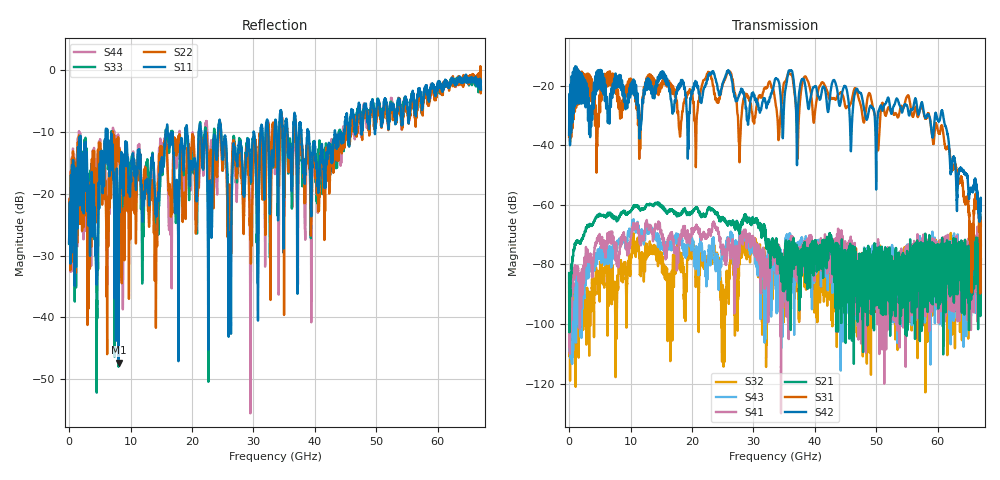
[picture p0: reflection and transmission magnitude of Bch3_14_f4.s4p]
!Agilent Technologies,N5247A,US51170199,A.09.90.13
!Agilent N5247A: A.09.90.13
!Date: Thursday, October 18, 2018 11:10:10
!Correction: S11(Full 4 Port(1,2,3,4))
!S12(Full 4 Port(1,2,3,4))
!S13(Full 4 Port(1,2,3,4))
!S14(Full 4 Port(1,2,3,4))
!S21(Full 4 Port(1,2,3,4))
!S22(Full 4 Port(1,2,3,4))
!S23(Full 4 Port(1,2,3,4))
!S24(Full 4 Port(1,2,3,4))
!S31(Full 4 Port(1,2,3,4))
!S32(Full 4 Port(1,2,3,4))
!S33(Full 4 Port(1,2,3,4))
!S34(Full 4 Port(1,2,3,4))
!S41(Full 4 Port(1,2,3,4))
!S42(Full 4 Port(1,2,3,4))
!S43(Full 4 Port(1,2,3,4))
!S44(Full 4 Port(1,2,3,4))
!S4P File: Measurements: <S11,S12,S13,S14>,
!<S21,S22,S23,S24>,
!<S31,S32,S33,S34>,
!<S41,S42,S43,S44>:
# Hz S  dB  R 50
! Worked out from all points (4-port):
!   6701 points, 10 MHz to 67 GHz, reference 50 ohm
!   strongest paths, dB at 10 MHz, 16.76 GHz, 33.51 GHz, 50.25 GHz, 67 GHz:
!     S42: -36.5, -28.1, -17.9, -29.7, -58.2
!     S31: -37.2, -21.6, -24.6, -41.7, -66.9
!     S21: -82.9, -61.6, -72.1, -93.5, -78.3
!     S41: -86.2, -69.8, -75.1, -92.1, -89.4
!     S43: -83.3, -72.1, -82.1, -80.5, -81.5
!     S32: -89.1, -85.5, -74.5, -82.3, -73.5
!   lowest |S11| = -47.3 dB at 8.049 GHz (marker M1), VSWR 1.01, Z = 50 + j0.431 ohm
!   |S11| at or under -10 dB: start of sweep to 5.976 GHz; 6.227 GHz to 15.72 GHz (9.489 GHz wide, 86.5 % of centre); 24.73 GHz to 30.02 GHz (5.288 GHz wide, 19.3 % of centre)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
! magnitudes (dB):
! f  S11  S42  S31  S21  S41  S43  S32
! 10 MHz  -28.0  -36.5  -37.2  -82.9  -86.2  -83.3  -89.1
! 8.049 GHz  -47.3  -18.5  -27.4  -64.4  -79.0  -72.2  -82.2
! 14.06 GHz  -22.8  -21.5  -21.3  -59.3  -66.4  -69.7  -76.3
! 15.57 GHz  -11.8  -16.2  -18.3  -61.8  -75.3  -73.5  -82.4
! 26.14 GHz  -27.2  -15.6  -15.4  -65.7  -75.3  -71.5  -80.8
! 55.1 GHz  -6.1  -27.6  -23.3  -81.3  -84.1  -91.6  -84.6
! 67 GHz  -3.1  -58.2  -66.9  -78.3  -89.4  -81.5  -73.5
